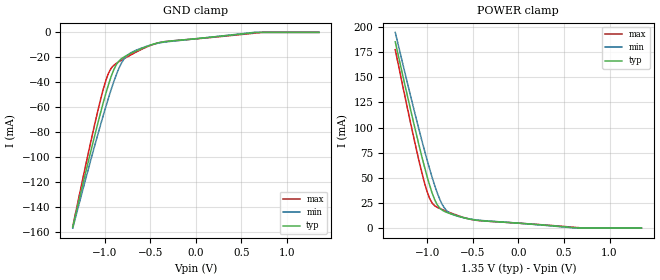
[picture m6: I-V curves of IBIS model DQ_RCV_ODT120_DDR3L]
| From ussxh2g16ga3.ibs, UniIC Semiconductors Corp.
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|   Model DQ_RCV_ODT120_DDR3L
[Model] DQ_RCV_ODT120_DDR3L
Model_type Input
Vinl =  0.540V
Vinh =  0.810V
C_comp   0.966pF   0.965pF   0.967pF
[Model Spec]
Vinh   0.810V   0.776V   0.860V
Vinl   0.540V   0.506V   0.590V
[Temperature Range]   25.000   95.000   -40.000
[Voltage Range]   1.350V   1.283V   1.450V
[GND_clamp]
|Voltage   I(typ)   I(min)   I(max)
-1.35V    -155.9mA   -156.8mA   -155.5mA
-1.126V   -87.57mA   -95.2mA    -79.03mA
-1.014V   -55.93mA   -66.14mA   -45.15mA
-958mV    -41.8mA    -52.49mA   -32.65mA
-930mV    -35.58mA   -46.03mA   -28.81mA
-874mV    -26.06mA   -34.24mA   -24.91mA
-818mV    -21.2mA    -24.88mA   -22.39mA
-762mV    -18.68mA   -19.05mA   -20.04mA
-706mV    -16.65mA   -16.06mA   -17.77mA
-370mV    -7.737mA   -8.076mA   -7.786mA
638mV     -251.5uA   -28.29uA   -660.9uA
1.35V     0A         0A         0A
[POWER_clamp]
|Voltage   I(typ)   I(min)   I(max)
-1.35V    185.2mA    194.6mA    177.4mA
-1.114V   91.62mA    106.7mA    76.53mA
-1.058V   70.97mA    87.02mA    55.03mA
-1.002V   51.7mA     68.15mA    36.61mA
-946mV    35.02mA    50.57mA    24.97mA
-890mV    23.28mA    35.15mA    20.71mA
-834mV    17.82mA    23.39mA    18.43mA
-778mV    15.41mA    16.65mA    16.39mA
-666mV    12.05mA    11.88mA    12.59mA
-414mV    7.452mA    7.708mA    7.336mA
650mV     229.5uA    0A         552.3uA
1.35V     0A         0A         0A
